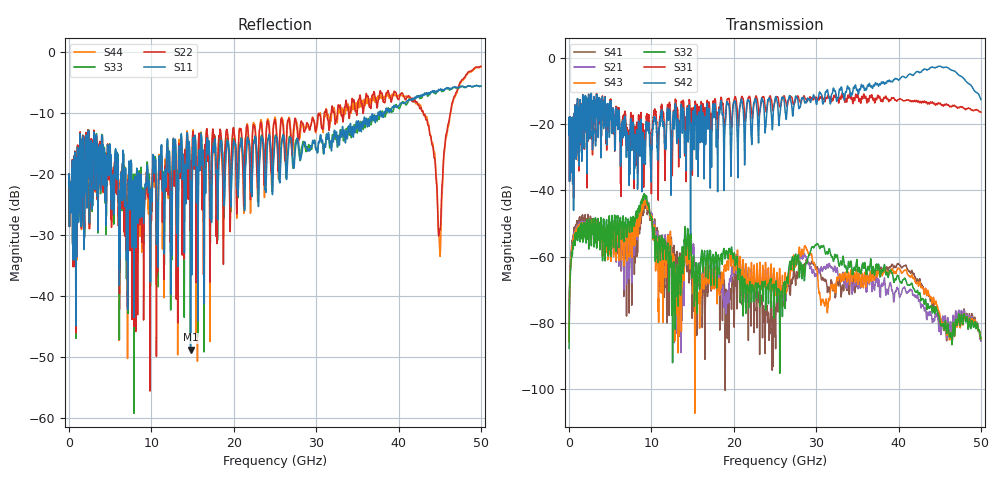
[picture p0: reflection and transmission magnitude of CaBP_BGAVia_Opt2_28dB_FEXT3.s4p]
!* Samtec Inc. NovaRay Examax Flyover System  *
!*  REV DATE  = 08/08/18  *
!*  TYPE  = TOUCHSTONE  *
!*  PORTS  = 4 port  *
!*  UNITS  = GHz  *
!*  DATA RANGE = DC  to 50 GHz; 10 MHz Step  *
!*  PARAMETER  = S  *
!*  FORMAT  = Real-Imaginary  *
!*  REFERENCE  = 50 ohms  *
!*  SOURCE  = HFSS  *
!*  VALIDATED  = No  *
!*  MANUFACTURER = SAMTEC  *
!*  INTERCONNECT = NVAx to EBCx to EBCx to NVAx  *
!*  [Full Channel NVAx to EBCx to EBCx to NVAx  with PCB Trace and BGA Via]  *
!*  BOUNDARY A  = Silicon BGA Ball Pad  *
!*  BOUNDARY B  = Silicon BGA Ball Pad  *
!*  NVAx (end a) ->>- (end b) NVAx  *
!*  Port 01 ->>- Port 02  *
!*  Port 03 ->>- Port 04  *
!***************************** CHANNEL MODEL ******************************************
# GHz S RI R 50
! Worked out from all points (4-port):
!   5000 points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, 10 MHz to 50 GHz, reference 50 ohm
!   strongest paths, dB at 10 MHz, 12.51 GHz, 25.01 GHz, 37.51 GHz, 50 GHz:
!     S42: -23.1, -25.0, -12.3, -8.2, -12.6
!     S31: -23.1, -28.5, -13.0, -11.3, -16.4
!     S32: -87.6, -71.7, -69.1, -63.7, -84.8
!     S43: -85.7, -59.8, -71.6, -64.6, -84.8
!     S21: -85.1, -65.4, -69.3, -68.8, -85.4
!     S41: -83.5, -58.5, -82.2, -63.9, -85.4
!   lowest |S11| = -48.8 dB at 14.75 GHz (marker M1), VSWR 1.01, Z = 49.7 - j0.221 ohm
!   |S11| at or under -10 dB: start of sweep to 37.51 GHz; 37.83997 GHz to 38.00552 GHz (165.6 MHz wide, 0.437 % of centre); 38.04261 GHz to 38.22467 GHz (182.1 MHz wide, 0.477 % of centre)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
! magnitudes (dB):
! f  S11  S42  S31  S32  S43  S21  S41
! 10 MHz  -22.1  -23.1  -23.1  -87.6  -85.7  -85.1  -83.5
! 9.23 GHz  -22.3  -29.2  -23.6  -41.7  -43.2  -42.6  -43.9
! 13.19 GHz  -22.9  -18.7  -15.6  -67.5  -69.1  -76.0  -61.3
! 14.75 GHz  -48.8  -53.1  -22.0  -53.9  -60.0  -55.0  -62.0
! 40.34 GHz  -8.4  -5.8  -12.5  -68.0  -64.8  -71.3  -63.3
! 44.98 GHz  -6.2  -2.5  -13.9  -78.7  -77.0  -80.7  -78.9
! 50 GHz  -5.6  -12.6  -16.4  -84.8  -84.8  -85.4  -85.4
